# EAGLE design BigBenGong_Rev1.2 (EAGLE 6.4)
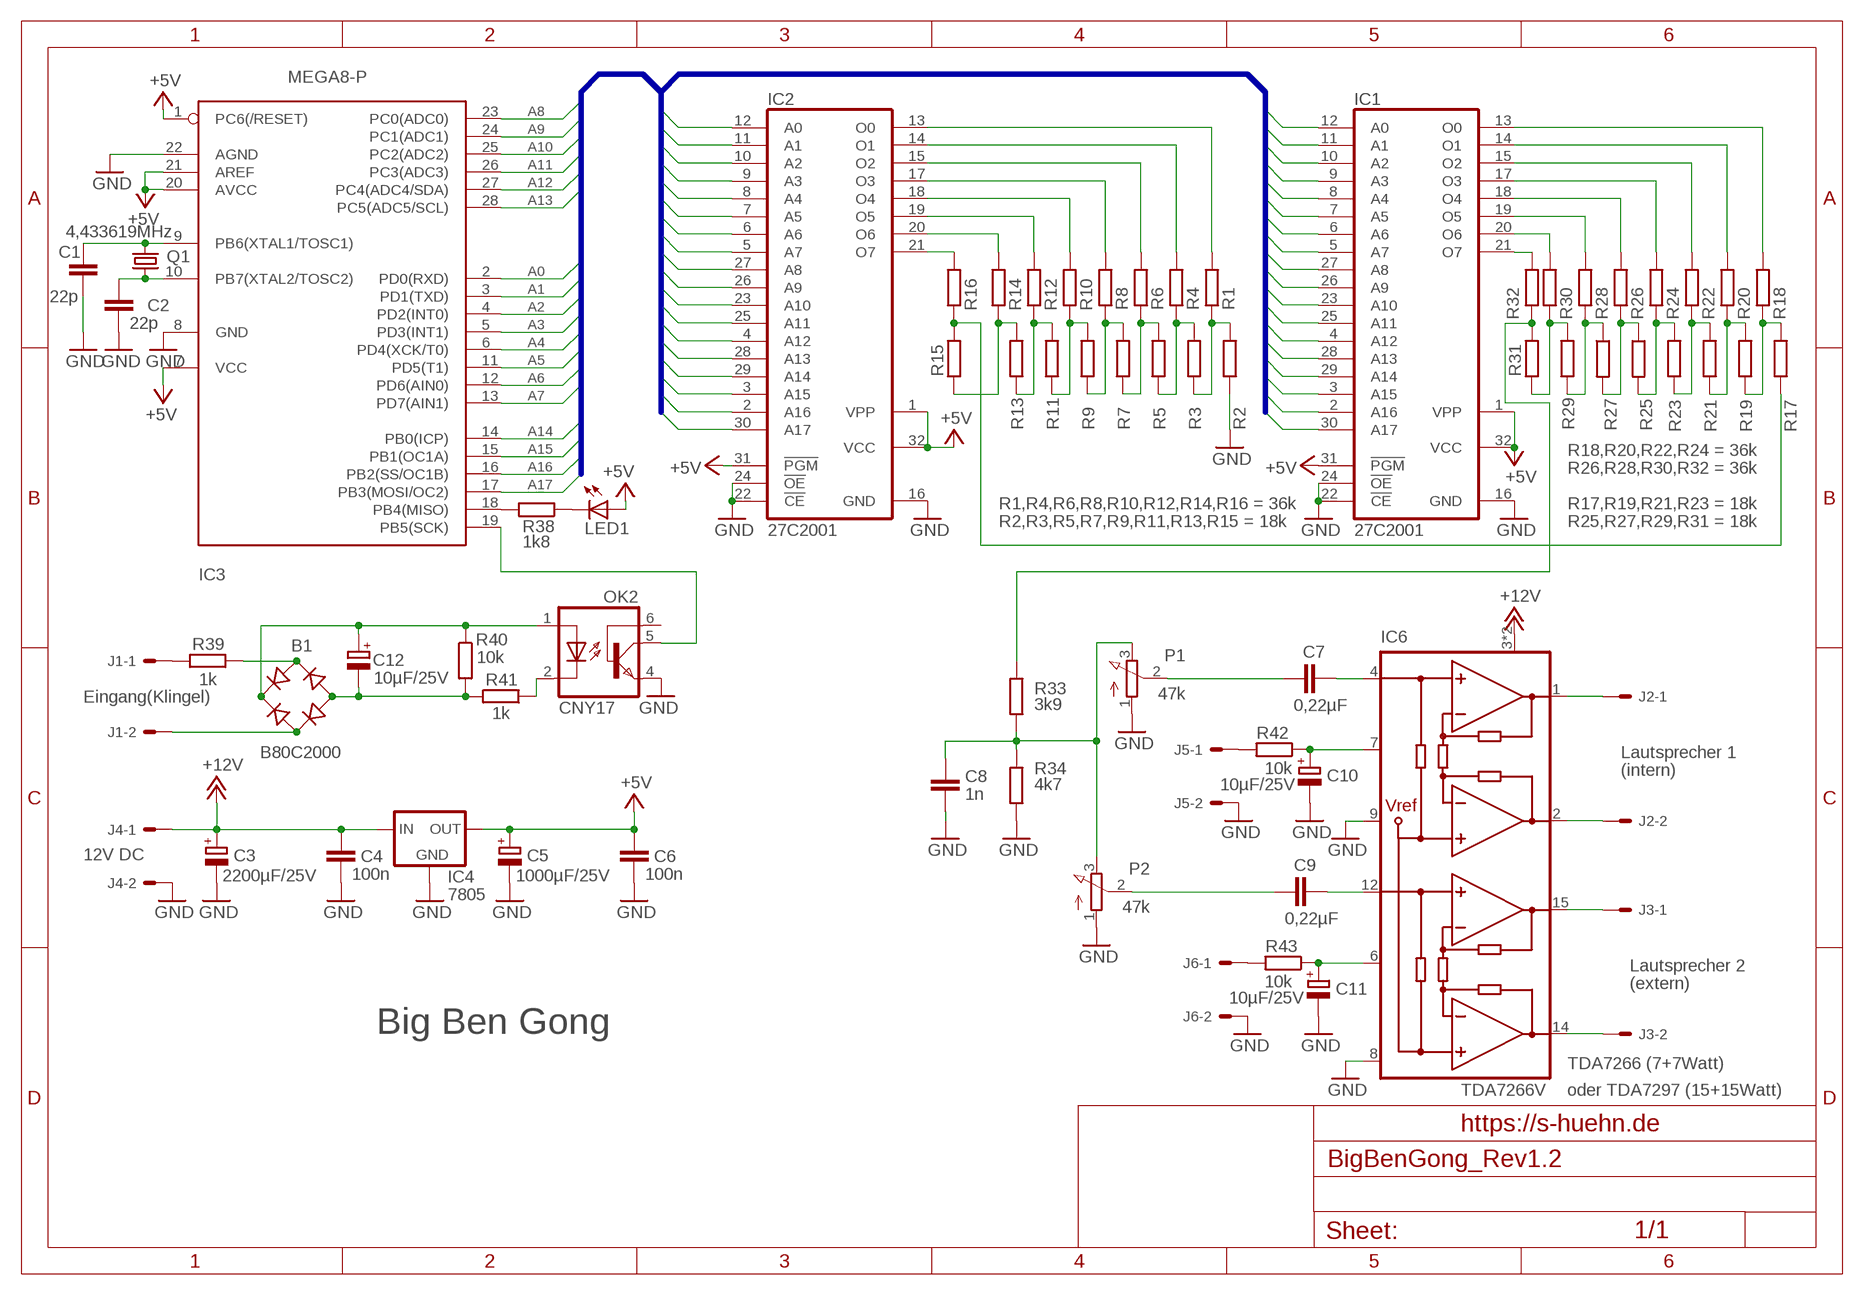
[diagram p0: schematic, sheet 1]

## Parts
B1  B80C2000  RB1A  [RB1A]
C1  22p  C-EU025-25X50A  [C025-025X050A]
C2  22p  C-EU025-25X50A  [C025-025X050A]
C3  2200µF/25V  CPOL-EUE7.5-16  [E7,5-16]
C4  100n  C-EU025-25X50A  [C025-025X050A]
C5  1000µF/25V  CPOL-EUE5-10.5  [E5-10,5]
C6  100n  C-EU025-25X50A  [C025-025X050A]
C7  0,22µF  C-EU025_050-035X075  [C025_050-035X075]
C8  1n  C-EU025-25X50A  [C025-025X050A]
C9  0,22µF  C-EU025_050-035X075  [C025_050-035X075]
C10  10µF/25V  CPOL-EUE2,5-6E  [E2,5-6E]
C11  10µF/25V  CPOL-EUE2,5-6E  [E2,5-6E]
C12  10µF/25V  CPOL-EUE2.5-6  [E2,5-6]
IC1  27C2001  27C2001D  [DIL32]
IC2  27C2001  27C2001D  [DIL32]
IC3  MEGA8-P  [DIL28-3]
IC4  7805  78XXS  [78XXS]
IC6  TDA7266V  [MULTIWATT15V]
J1  22-27-2021-02  [6410-02]
J2  22-27-2021-02  [6410-02]
J3  22-27-2021-02  [6410-02]
J4  22-27-2021-02  [6410-02]
J5  22-27-2021-02  [6410-02]
J6  22-27-2021-02  [6410-02]
LED1  LED5MM_MOLEX_S  [6410-02]
OK2  CNY17  [DIL06]
P1  47k  POTIMOL-H  [6410-03]
P2  47k  POTIMOL-H  [6410-03]
Q1  4,433619MHz  CRYSTALHC49U-V  [HC49U-V]
R1  R-EU_0207/10A  [0207/10A]
R2  R-EU_0207/10A  [0207/10A]
R3  R-EU_0207/10A  [0207/10A]
R4  R-EU_0207/10A  [0207/10A]
R5  R-EU_0207/10A  [0207/10A]
R6  R-EU_0207/10A  [0207/10A]
R7  R-EU_0207/10A  [0207/10A]
R8  R-EU_0207/10A  [0207/10A]
R9  R-EU_0207/10A  [0207/10A]
R10  R-EU_0207/10A  [0207/10A]
R11  R-EU_0207/10A  [0207/10A]
R12  R-EU_0207/10A  [0207/10A]
R13  R-EU_0207/10A  [0207/10A]
R14  R-EU_0207/10A  [0207/10A]
R15  R-EU_0207/10A  [0207/10A]
R16  R-EU_0207/10A  [0207/10A]
R17  R-EU_0207/10A  [0207/10A]
R18  R-EU_0207/10A  [0207/10A]
R19  R-EU_0207/10A  [0207/10A]
R20  R-EU_0207/10A  [0207/10A]
R21  R-EU_0207/10A  [0207/10A]
R22  R-EU_0207/10A  [0207/10A]
R23  R-EU_0207/10A  [0207/10A]
R24  R-EU_0207/10A  [0207/10A]
R25  R-EU_0207/10A  [0207/10A]
R26  R-EU_0207/10A  [0207/10A]
R27  R-EU_0207/10A  [0207/10A]
R28  R-EU_0207/10A  [0207/10A]
R29  R-EU_0207/10A  [0207/10A]
R30  R-EU_0207/10A  [0207/10A]
R31  R-EU_0207/10A  [0207/10A]
R32  R-EU_0207/10A  [0207/10A]
R33  3k9  R-EU_0207/10A  [0207/10A]
R34  4k7  R-EU_0207/10A  [0207/10A]
R38  1k8  R-EU_0207/10A  [0207/10A]
R39  1k  R-EU_0207/10A  [0207/10A]
R40  10k  R-EU_0207/10A  [0207/10A]
R41  1k  R-EU_0207/10A  [0207/10A]
R42  10k  R-EU_0207/10A  [0207/10A]
R43  10k  R-EU_0207/10A  [0207/10A]

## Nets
+5V: C5.+ C6.1 IC1.1(VPP) IC1.31(!PGM) IC1.32(VCC) IC2.1(VPP) IC2.31(!PGM) IC2.32(VCC) IC3.1(PC6(/RESET)) IC3.7(VCC) IC3.20(AVCC) IC3.21(AREF) IC4.OUT LED1.A
+12V: C3.+ C4.1 IC4.IN IC6.3(VCC) IC6.13(VCC) J4.1
A0: IC1.12(A0) IC2.12(A0) IC3.2(PD0(RXD))
A1: IC1.11(A1) IC2.11(A1) IC3.3(PD1(TXD))
A2: IC1.10(A2) IC2.10(A2) IC3.4(PD2(INT0))
A3: IC1.9(A3) IC2.9(A3) IC3.5(PD3(INT1))
A4: IC1.8(A4) IC2.8(A4) IC3.6(PD4(XCK/T0))
A5: IC1.7(A5) IC2.7(A5) IC3.11(PD5(T1))
A6: IC1.6(A6) IC2.6(A6) IC3.12(PD6(AIN0))
A7: IC1.5(A7) IC2.5(A7) IC3.13(PD7(AIN1))
A8: IC1.27(A8) IC2.27(A8) IC3.23(PC0(ADC0))
A9: IC1.26(A9) IC2.26(A9) IC3.24(PC1(ADC1))
A10: IC1.23(A10) IC2.23(A10) IC3.25(PC2(ADC2))
A11: IC1.25(A11) IC2.25(A11) IC3.26(PC3(ADC3))
A12: IC1.4(A12) IC2.4(A12) IC3.27(PC4(ADC4/SDA))
A13: IC1.28(A13) IC2.28(A13) IC3.28(PC5(ADC5/SCL))
A14: IC1.29(A14) IC2.29(A14) IC3.14(PB0(ICP))
A15: IC1.3(A15) IC2.3(A15) IC3.15(PB1(OC1A))
A16: IC1.2(A16) IC2.2(A16) IC3.16(PB2(SS/OC1B))
A17: IC1.30(A17) IC2.30(A17) IC3.17(PB3(MOSI/OC2))
GND: C1.2 C2.2 C3.- C4.2 C5.- C6.2 C8.2 C10.- C11.- IC1.16(GND) IC1.22(!CE) IC1.24(!OE) IC2.16(GND) IC2.22(!CE) IC2.24(!OE) IC3.8(GND) IC3.22(AGND) IC4.GND IC6.8(PW-GND) IC6.9(S-GND) J4.2 J5.2 J6.2 OK2.4(EMI) P1.1(A) P2.1(A) R2.1 R34.2
N$1: IC2.13(O0) R1.1
N$2: IC2.14(O1) R4.1
N$3: IC2.17(O3) R8.1
N$4: IC2.18(O4) R10.1
N$5: IC2.15(O2) R6.1
N$6: IC2.19(O5) R12.1
N$7: IC2.20(O6) R14.1
N$8: IC2.21(O7) R16.1
N$9: IC1.13(O0) R18.1
N$10: IC1.14(O1) R20.1
N$11: IC1.15(O2) R22.1
N$12: IC1.17(O3) R24.1
N$13: IC1.18(O4) R26.1
N$14: IC1.19(O5) R28.1
N$15: IC1.20(O6) R30.1
N$16: IC1.21(O7) R32.1
N$17: B1.+ C12.+ OK2.1(A) R40.1
N$18: R29.2 R30.2 R31.1
N$19: R27.1 R28.2 R29.1
N$20: R25.1 R26.2 R27.2
N$21: R23.2 R24.2 R25.2
N$22: R21.2 R22.2 R23.1
N$23: R19.2 R20.2 R21.1
N$24: R17.2 R18.2 R19.1
N$25: R15.2 R16.2 R17.1
N$26: R13.2 R14.2 R15.1
N$27: C1.1 IC3.9(PB6(XTAL1/TOSC1)) Q1.2
N$28: R11.2 R12.2 R13.1
N$29: C2.1 IC3.10(PB7(XTAL2/TOSC2)) Q1.1
N$30: R9.2 R10.2 R11.1
N$31: R7.2 R8.2 R9.1
N$32: R5.2 R6.2 R7.1
N$33: R3.2 R4.2 R5.1
N$34: R1.2 R2.2 R3.1
N$35: IC3.18(PB4(MISO)) R38.2
N$36: IC3.19(PB5(SCK)) OK2.5(COL)
N$37: OK2.2(C) R41.1
N$38: B1.- C12.- R40.2 R41.2
N$41: C7.1 IC6.4(IN1)
N$42: R31.2 R32.2 R33.1
N$43: LED1.C R38.1
N$44: J1.1 R39.1
N$45: B1.AC2 J1.2
N$46: IC6.1(OUT1+) J2.1
N$47: IC6.2(OUT1-) J2.2
N$48: IC6.15(OUT2+) J3.1
N$49: IC6.14(OUT2-) J3.2
N$50: C9.1 IC6.12(IN2)
N$51: B1.AC1 R39.2
N$52: C10.+ IC6.7(ST-BY) R42.1
N$53: C11.+ IC6.6(MUTE) R43.1
N$54: J5.1 R42.2
N$55: J6.1 R43.2
N$56: C7.2 C7.3 P1.2(S)
N$57: C9.2 C9.3 P2.2(S)
N$58: C8.1 P1.3(E) P2.3(E) R33.2 R34.1
Unconnected: OK2.6(BAS)

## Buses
A[0..17]

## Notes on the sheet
- R18,R20,R22,R24 = 36k
- R26,R28,R30,R32 = 36k
- R1,R4,R6,R8,R10,R12,R14,R16 = 36k | R17,R19,R21,R23 = 18k
- R2,R3,R5,R7,R9,R11,R13,R15 = 18k | R25,R27,R29,R31 = 18k
- Eingang(Klingel)
- Lautsprecher 1
- (intern)
- 12V DC
- Lautsprecher 2
- (extern)
- Big Ben Gong
- TDA7266 (7+7Watt)
- oder TDA7297 (15+15Watt)
- https://s-huehn.de

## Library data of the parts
B1 = rectifier:RB1A: RECTIFIER 1 A
C1 C2 C4 C6-C9 = rcl:C-EU: CAPACITOR, European symbol
C3 C5 C10-C12 = rcl:CPOL-EU: POLARIZED CAPACITOR, European symbol
IC1 IC2 = memory-nec:27C2001D: MEMORY
IC3 = avr-7:MEGA8-P: MICROCONTROLLER 8 Kbytes FLASH 1 kbytes SRAM 512 bytes EEPROM USART 4-channel 10 bit ADC 2-channel 8 bit ADC
IC4 = v-reg:78XXS: VOLTAGE REGULATOR
IC6 = sgs-thom:TDA7266
J1-J6 = con-molex:22-?-02: CONNECTOR
LED1 = led:LED: LED
OK2 = optocoupler-2:CNY17: SIEMENS OPTO COUPLER
P1 P2 = pot:POTI
Q1 = crystal:CRYSTAL: CRYSTAL
R1-R34 R38-R43 = rcl:R-EU_: RESISTOR, European symbol

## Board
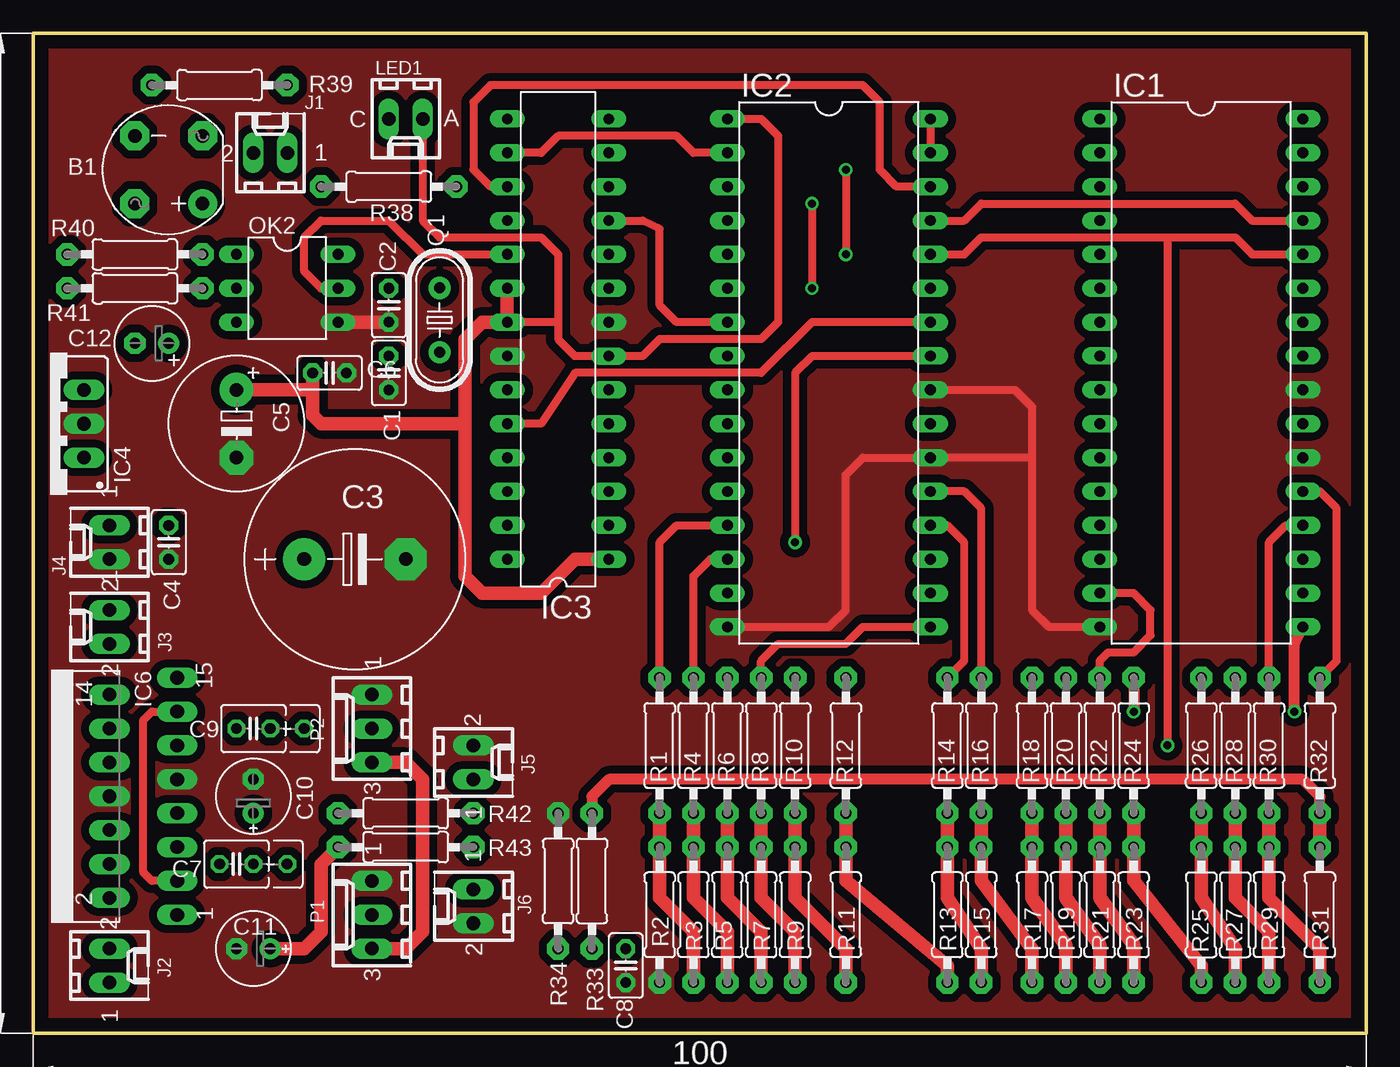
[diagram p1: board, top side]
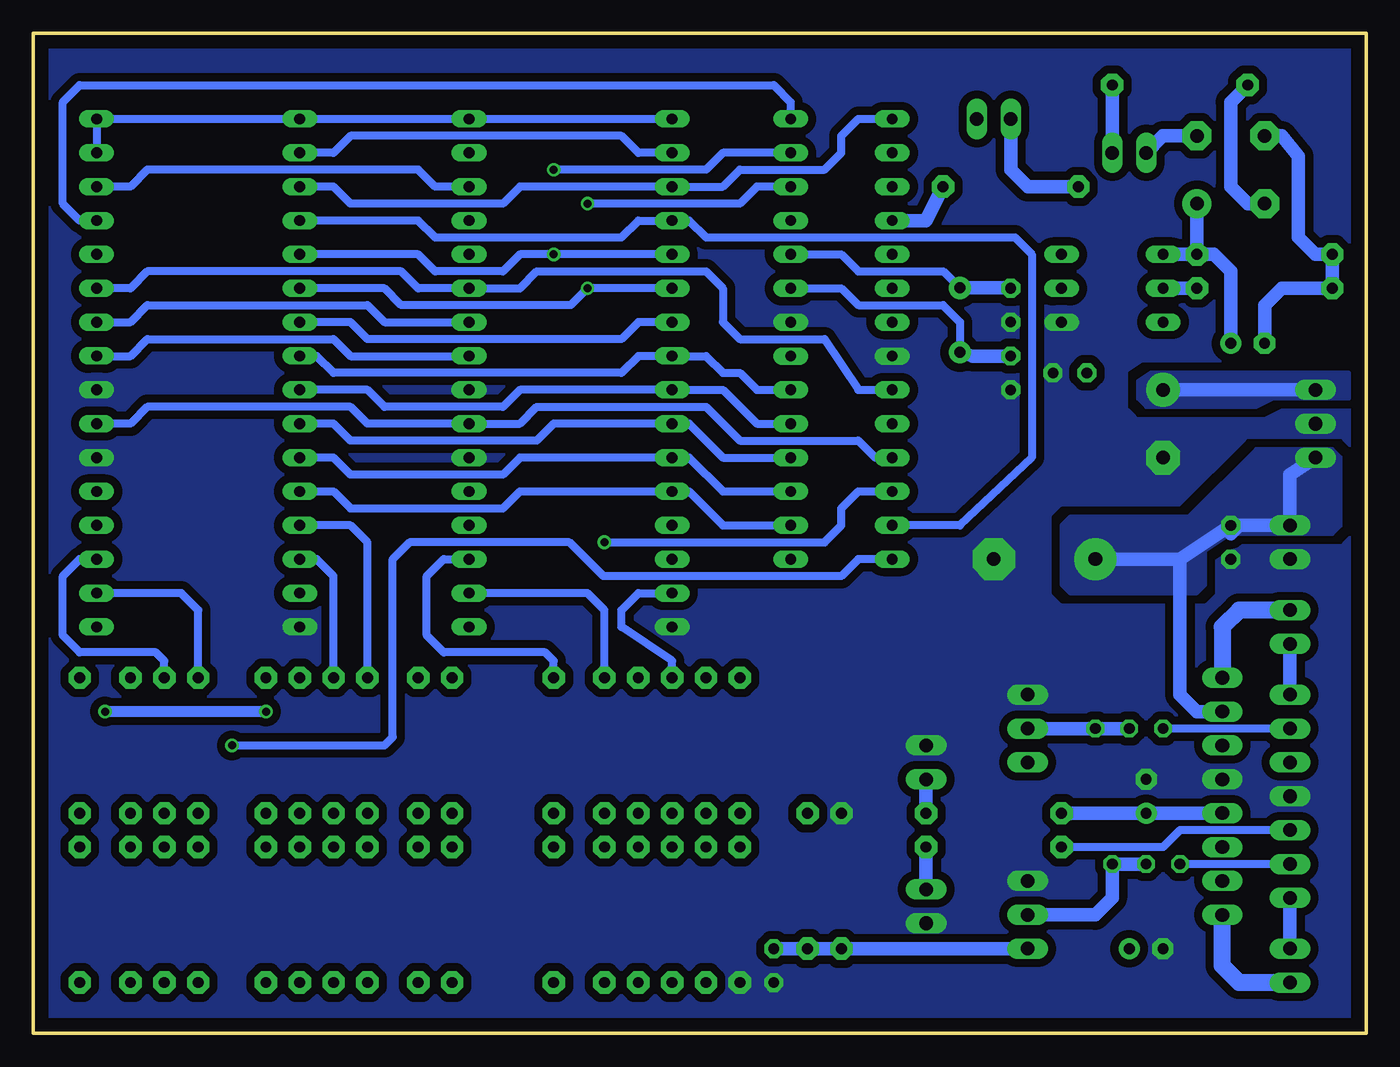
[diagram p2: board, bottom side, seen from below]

Size 100 x 75 mm. Coordinates in mm from the lower left corner, seen from the top.
Outline: 0,0 100,0 100,75 0,75 0,0
Copper layers (1*16): Top 0.035mm / dielectric 1.5mm / Bottom 0.035mm
Design rules "default *": minimum track width 10mil, minimum drill 0.2mm, track to track 8mil, track to pad 8mil, pad to pad 8mil, via to via 8mil, smd to smd 8mil, copper to edge 40mil, drill to drill 8mil, minimum pad ring 10mil, minimum via ring 8mil, stop-mask expansion 4mil, vias tented up to drill 0mil, thermal gap 10mil

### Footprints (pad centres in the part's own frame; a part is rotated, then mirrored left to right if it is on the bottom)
RB1A = drill 1.016 pad 2.184: + -2.54,2.54 | drill 1.016 pad 2.184 octagon: - 2.54,-2.54; AC1 2.54,2.54; AC2 -2.54,-2.54
C025-025X050A = drill 0.8 pad 1.422 octagon: 1 -1.27,0; 2 1.27,0
E7,5-16 = drill 1.016 pad 3.15: + -3.81,0 | drill 1.016 pad 3.15 octagon: - 3.81,0
E5-10,5 = drill 1.016 pad 2.54: + -2.54,0 | drill 1.016 pad 2.54 octagon: - 2.54,0
C025_050-035X075 = drill 0.813 octagon: 1 -1.27,0; 2 1.27,0; 3 3.81,0
E2,5-6E = drill 0.813 pad 1.575: + -1.27,0 | drill 0.813 pad 1.575 octagon: - 1.27,0
E2,5-6 = drill 0.813 pad 1.6: + -1.27,0 | drill 0.813 pad 1.6 octagon: - 1.27,0
DIL32 = drill 0.813 long: 1 -19.05,-7.62; 2 -16.51,-7.62; 3 -13.97,-7.62; 4 -11.43,-7.62; 5 -8.89,-7.62; 6 -6.35,-7.62; 7 -3.81,-7.62; 8 -1.27,-7.62; 9 1.27,-7.62; 10 3.81,-7.62; 11 6.35,-7.62; 12 8.89,-7.62; 13 11.43,-7.62; 14 13.97,-7.62; 15 16.51,-7.62; 16 19.05,-7.62; 17 19.05,7.62; 18 16.51,7.62; 19 13.97,7.62; 20 11.43,7.62; 21 8.89,7.62; 22 6.35,7.62; 23 3.81,7.62; 24 1.27,7.62; 25 -1.27,7.62; 26 -3.81,7.62; 27 -6.35,7.62; 28 -8.89,7.62; 29 -11.43,7.62; 30 -13.97,7.62; 31 -16.51,7.62; 32 -19.05,7.62
DIL28-3 = drill 0.813 long: 1 -16.51,-3.81; 2 -13.97,-3.81; 3 -11.43,-3.81; 4 -8.89,-3.81; 5 -6.35,-3.81; 6 -3.81,-3.81; 7 -1.27,-3.81; 8 1.27,-3.81; 9 3.81,-3.81; 10 6.35,-3.81; 11 8.89,-3.81; 12 11.43,-3.81; 13 13.97,-3.81; 14 16.51,-3.81; 15 16.51,3.81; 16 13.97,3.81; 17 11.43,3.81; 18 8.89,3.81; 19 6.35,3.81; 20 3.81,3.81; 21 1.27,3.81; 22 -1.27,3.81; 23 -3.81,3.81; 24 -6.35,3.81; 25 -8.89,3.81; 26 -11.43,3.81; 27 -13.97,3.81; 28 -16.51,3.81
78XXS = drill 1.016 long: GND 0,-2.54; IN -2.54,-2.54; OUT 2.54,-2.54
MULTIWATT15V = drill 1.016 long: 1 -8.89,-7.62; 2 -7.62,-2.54; 3 -6.35,-7.62; 4 -5.08,-2.54; 5 -3.81,-7.62; 6 -2.54,-2.54; 7 -1.27,-7.62; 8 0,-2.54; 9 1.27,-7.62; 10 2.54,-2.54; 11 3.81,-7.62; 12 5.08,-2.54; 13 6.35,-7.62; 14 7.62,-2.54; 15 8.89,-7.62
6410-02 = drill 1.016 long: 1 1.27,0; 2 -1.27,0
6410-02' = drill 1.016 long: A -1.27,0; C 1.27,0
DIL06 = drill 0.813 long: 1 -2.54,-3.81; 2 0,-3.81; 3 2.54,-3.81; 4 2.54,3.81; 5 0,3.81; 6 -2.54,3.81
6410-03 = drill 1.016 long: 1 2.54,0; 2 0,0; 3 -2.54,0
HC49U-V = drill 0.813 pad 1.676: 1 -2.413,0; 2 2.413,0
0207/10A = drill 0.813 pad 1.676 octagon: 1 -5.08,0; 2 5.08,0

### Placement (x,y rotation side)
B1  10.16,64.77 180 top
C1  26.67,49.53 270 top
C2  26.67,54.61 270 top
C3  24.13,35.56 0 top
C4  10.16,36.83 270 top
C5  15.24,45.72 270 top
C6  22.23,49.53 0 top
C7  15.24,12.7 0 top
C8  44.45,5.08 270 top
C9  16.51,22.86 0 top
C10  16.51,17.78 90 top
C11  16.51,6.35 180 top
C12  8.89,51.75 180 top
IC1  87.63,49.53 270 top
IC2  59.69,49.53 270 top
IC3  39.37,52.07 90 top
IC4  1.27,45.72 90 top
IC6  3.17,17.78 90 top
J1  17.78,66.04 0 top
J2  5.71,5.08 270 top
J3  5.71,30.48 90 top
J4  5.71,36.83 90 top
J5  33.02,20.32 270 top
J6  33.02,9.53 90 top
LED1  [6410-02']  27.94,68.58 180 top
OK2  19.05,55.88 270 top
P1  25.4,8.89 90 top
P2  25.4,22.86 90 top
Q1  30.48,53.5 270 top
R1  46.99,21.59 270 top
R2  46.99,8.89 90 top
R3  49.53,8.89 90 top
R4  49.53,21.59 270 top
R5  52.07,8.89 90 top
R6  52.07,21.59 270 top
R7  54.61,8.89 90 top
R8  54.61,21.59 270 top
R9  57.15,8.89 90 top
R10  57.15,21.59 270 top
R11  60.96,8.89 90 top
R12  60.96,21.59 270 top
R13  68.58,8.89 90 top
R14  68.58,21.59 270 top
R15  71.12,8.89 90 top
R16  71.12,21.59 270 top
R17  74.93,8.89 90 top
R18  74.93,21.59 270 top
R19  77.47,8.89 90 top
R20  77.47,21.59 270 top
R21  80.01,8.89 90 top
R22  80.01,21.59 270 top
R23  82.55,8.89 90 top
R24  82.55,21.59 270 top
R25  87.63,8.89 270 top
R26  87.63,21.59 270 top
R27  90.17,8.89 270 top
R28  90.17,21.59 270 top
R29  92.71,8.89 90 top
R30  92.71,21.59 270 top
R31  96.52,8.89 90 top
R32  96.52,21.59 270 top
R33  41.91,11.43 270 top
R34  39.37,11.43 90 top
R38  26.67,63.5 0 top
R39  13.97,71.12 180 top
R40  7.62,58.42 180 top
R41  7.62,55.88 180 top
R42  27.94,16.51 0 top
R43  27.94,13.97 0 top

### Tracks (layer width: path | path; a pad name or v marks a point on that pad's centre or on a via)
+5V
  Top 0.61: IC2.32 IC2.31 | IC2.1 54.61,68.58 55.88,67.31 55.88,53.34 54.61,52.07 46.99,52.07 45.72,50.8 IC3.7 40.64,50.8 39.37,52.07 39.37,53.34 | 39.37,53.34 IC3.21 | LED1.A 29.21,60.96 30.48,59.69 38.1,59.69 39.37,58.42 39.37,53.34
  Top 1.016: IC3.20 IC3.21 33.66,53.34 32.38,52.07 32.38,45.72 | 32.38,45.72 32.38,34.29 33.66,33.02 38.1,33.02 40.64,35.56 IC3.1 | 32.38,45.72 21.59,45.72 20.95,46.35 20.95,48.26 | 20.95,48.26 C5.+ | C6.1 20.95,48.26
  Bottom 0.61: IC2.1 IC2.32 IC1.1 IC1.32 IC1.31
  Bottom 1.016: IC4.OUT C5.+
  pour Bottom (rank 2, no thermals): 1.27,49.53 16.19,49.53 17.14,48.9 17.14,47.62 16.51,46.99 8.26,46.99 6.99,47.62 1.27,47.62
+12V
  Top 0.61: IC6.3 8.89,11.43 8.26,12.06 8.26,23.5 8.89,24.13 IC6.13
  Bottom 1.016: IC4.IN 5.71,41.91 J4.1 9.53,38.1 10.16,37.47 C4.1 13.97,35.56 | 13.97,35.56 13.97,25.4 12.7,24.13 IC6.13 | C3.+ 13.97,35.56
  pour Bottom (rank 2, no thermals): 2.54,43.81 8.26,43.81 13.34,38.73 22.23,38.73 22.86,38.1 22.86,33.66 22.23,33.02 12.7,33.02 12.06,33.66 12.06,36.2 10.16,37.47 2.54,37.47 1.91,38.1 1.91,43.18
A0
  Bottom 0.254: IC2.12 50.8,40.64
  Bottom 0.61: IC2.12 63.5,40.64 64.77,39.37 76.2,39.37 77.47,40.64 IC1.12 | 50.8,40.64 48.26,38.1 IC3.2
A1
  Bottom 0.61: IC3.3 48.26,40.64 50.8,43.18 IC2.11 63.5,43.18 64.77,41.91 76.2,41.91 77.47,43.18 IC1.11
A2
  Bottom 0.254: IC2.10 50.8,45.72
  Bottom 0.61: IC3.4 48.26,43.18 50.8,45.72 | IC1.10 77.47,45.72 76.2,44.45 62.23,44.45 60.96,45.72 IC2.10
A3
  Bottom 0.61: IC1.9 74.93,48.26 73.66,46.99 64.77,46.99 63.5,48.26 IC2.9 48.26,48.26 45.72,45.72 IC3.5
A4
  Bottom 0.61: IC1.8 78.74,50.8 77.47,49.53 55.88,49.53 54.61,50.8 IC2.8 49.53,50.8 48.26,49.53 46.99,49.53 45.72,48.26 IC3.6
A5
  Top 0.61: IC3.11 45.72,60.96 46.99,60.33 46.99,54.61 48.26,53.34 IC2.7
  Bottom 0.61: IC1.7 76.2,53.34 74.93,52.07 55.88,52.07 54.61,53.34 IC2.7
A6  (via drill 0.6)
  Top 0.61: v58.42,62.23 v58.42,55.88
  Bottom 0.61: IC1.6 73.66,55.88 72.39,54.61 59.69,54.61 v58.42,55.88 IC2.6 | IC3.12 45.72,63.5 46.99,62.23 v58.42,62.23
A7  (via drill 0.6)
  Top 0.61: v60.96,64.77 v60.96,58.42
  Bottom 0.61: IC1.5 71.12,58.42 69.85,57.15 64.77,57.15 63.5,58.42 v60.96,58.42 IC2.5 | IC3.13 48.26,66.04 49.53,64.77 v60.96,64.77
A8
  Bottom 0.61: IC1.27 92.71,55.88 91.44,57.15 72.39,57.15 71.12,55.88 IC2.27 63.5,55.88 62.23,57.15 49.53,57.15 48.26,55.88 48.26,53.34 46.99,52.07 40.64,52.07 38.1,48.26 IC3.23
A9
  Top 0.61: IC3.24 38.1,45.72 40.64,49.53 54.61,49.53 58.42,53.34 IC2.26
  Bottom 0.61: IC2.26 73.66,53.34 74.93,54.61 91.44,54.61 92.71,53.34 IC1.26
A10
  Bottom 0.61: IC3.25 36.83,43.18 38.1,44.45 46.99,44.45 49.53,46.99 62.23,46.99 63.5,45.72 IC2.23 74.93,45.72 76.2,46.99 91.44,46.99 92.71,45.72 IC1.23
A11  (via drill 0.61)
  Top 0.61: v57.15,36.83 57.15,49.53 58.42,50.8 IC2.25
  Bottom 0.61: IC2.25 76.2,50.8 77.47,52.07 91.44,52.07 92.71,50.8 IC1.25 | IC3.26 38.1,40.64 39.37,39.37 39.37,38.1 40.64,36.83 v57.15,36.83
A12
  Bottom 0.61: IC1.4 71.12,60.96 69.85,59.69 55.88,59.69 54.61,60.96 IC2.4 50.8,60.96 49.53,59.69 26.35,59.69 25.08,58.42 25.08,43.18 30.48,38.1 IC3.27
A13  (via drill 0.6)
  Top 0.61: IC1.28 91.44,58.42 90.17,59.69 85.09,59.69 | IC2.28 69.85,58.42 71.12,59.69 85.09,59.69 | 85.09,59.69 v85.09,21.59
  Bottom 0.61: IC3.28 38.1,35.56 39.37,34.29 57.23,34.29 59.77,36.83 71.75,36.83 73.03,35.56 73.03,22.23 73.66,21.59 v85.09,21.59
A14
  Top 0.61: IC1.29 91.44,60.96 90.17,62.23 71.12,62.23 69.85,60.96 IC2.29
  Bottom 0.61: IC3.14 43.18,69.85 44.45,71.12 96.52,71.12 97.79,69.85 97.79,62.23 96.52,60.96 IC1.29
A15
  Bottom 0.61: IC1.3 77.47,63.5 76.2,62.23 64.77,62.23 63.5,63.5 IC2.3 48.26,63.5 46.99,64.77 40.64,64.77 39.37,66.04 39.37,67.31 38.1,68.58 IC3.15
A16
  Top 0.61: IC3.16 38.1,66.04 39.37,67.31 48.26,67.31 49.53,66.04 IC2.2
  Bottom 0.61: IC1.2 77.47,66.04 76.2,67.31 55.88,67.31 54.61,66.04 IC2.2
A17
  Top 0.61: IC3.17 34.29,63.5 33.02,64.77 33.02,69.85 34.29,71.12 62.23,71.12 63.5,69.85 63.5,64.77 64.77,63.5 IC2.30
  Bottom 0.254: IC2.30 68.58,63.5
  Bottom 0.61: IC1.30 92.71,63.5 91.44,64.77 71.12,64.77 69.85,63.5 68.58,63.5
GND
  Top 0.61: IC2.24 73.66,48.26 74.93,46.99 74.93,43.18 | 74.93,43.18 IC2.22 62.23,43.18 60.96,41.91 60.96,31.75 59.69,30.48 IC2.16 | 74.93,43.18 74.93,31.75 76.2,30.48 IC1.16
  Top 1.016: OK2.4 C2.2
  Bottom 0.254: IC2.22
  pour Top (isolate 0.61, no thermals): 0,0 100,0 100,2 100,75 0,75 0,64
  pour Bottom (isolate 0.61, rank 6, no thermals): 0,0 100,0 100,2 100,75 0,75 0,71
N$1
  Top 0.61: IC2.13 48.26,38.1 46.99,36.83 R1.1
N$2
  Top 0.61: IC2.14 50.8,35.56 49.53,34.29 R4.1
N$3
  Top 0.61: IC2.17 62.23,30.48 60.96,29.21 55.88,29.21 54.61,27.94 R8.1
N$4
  Bottom 0.61: IC2.18 58.42,33.02 57.15,31.75 R10.1
N$5
  Bottom 0.61: IC2.15 54.61,33.02 55.88,31.75 55.88,30.48 52.07,27.94 R6.1
N$6
  Bottom 0.61: IC2.19 69.22,35.56 70.48,34.29 70.48,29.84 69.22,28.57 61.59,28.57 60.96,27.94 R12.1
N$7
  Top 0.61: IC2.20 68.58,38.1 69.85,36.83 69.85,27.94 R14.1
N$8
  Top 0.61: IC2.21 69.85,40.64 71.12,39.37 R16.1
N$9
  Bottom 0.61: IC1.13 76.2,38.1 74.93,36.83 R18.1
N$10
  Bottom 0.61: IC1.14 78.74,35.56 77.47,34.29 R20.1
N$11
  Top 0.61: IC1.15 82.55,33.02 83.82,31.75 83.82,29.84 82.55,28.57 80.64,28.57 80.01,27.94 R22.1
N$12  (via drill 0.6)
  Top 0.813: v94.61,24.13 94.61,29.21 IC1.17 | R24.1 v82.55,24.13
  Bottom 0.813: v82.55,24.13 v94.61,24.13
N$13
  Bottom 0.61: IC1.18 88.9,33.02 87.63,31.75 R26.1
N$14
  Bottom 0.61: IC1.19 96.52,35.56 97.79,34.29 97.79,29.84 96.52,28.57 90.81,28.57 90.17,27.94 R28.1
N$15
  Top 0.61: IC1.20 93.98,38.1 92.71,36.83 R30.1
N$16
  Top 0.61: IC1.21 96.52,40.64 97.79,39.37 97.79,27.94 R32.1
N$17
  Bottom 1.016: B1.+ R40.1 | R40.1 OK2.1 | C12.+ 10.16,57.15 11.43,58.42 R40.1
N$18
  Top 1.016: R30.2 R29.2 92.71,10.16 96.52,6.35 R31.1
N$19
  Top 1.016: R28.2 R27.1 90.17,10.16 92.71,7.62 R29.1
N$20
  Top 1.016: R26.2 R25.1 87.63,10.16 90.17,6.35 R27.2
N$21
  Top 1.016: R24.2 R23.2 82.55,11.43 87.63,5.08 R25.2
N$22
  Top 1.016: R22.2 R21.2 80.01,10.16 82.55,6.62 R23.1
N$23
  Top 1.016: R20.2 R19.2 77.47,10.16 80.01,6.62 R21.1
N$24
  Top 1.016: R18.2 R17.2 74.93,10.16 77.47,6.62 R19.1
N$25
  Top 1.016: R16.2 R15.2 71.12,11.43 74.93,6.35 R17.1
N$26
  Top 1.016: R14.2 R13.2 68.58,10.16 71.12,6.35 R15.1
N$27
  Bottom 0.61: IC3.9 39.37,55.88 38.1,54.61 31.75,54.61 30.48,53.34 Q1.2
  Bottom 1.016: Q1.2 29.49,50.77 C1.1
N$28
  Top 1.016: R12.2 R11.2 60.96,11.43 68.58,5.08 R13.1
N$29
  Bottom 0.61: 26.7,55.91 C2.1 | IC3.10 39.37,58.42 38.1,57.15 31.72,57.15 Q1.1
  Bottom 1.016: Q1.1 26.7,55.91
N$30
  Top 1.016: R10.2 R9.2 57.15,10.16 60.96,6.35 R11.1
N$31
  Top 1.016: R8.2 R7.2 54.61,10.16 57.15,7.62 R9.1
N$32
  Top 1.016: R6.2 R5.2 52.07,10.16 54.61,7.62 R7.1
N$33
  Top 1.016: R4.2 R3.2 49.53,10.16 52.07,7.62 R5.1
N$34
  Top 1.016: R1.2 R2.2 46.99,10.16 49.53,7.62 R3.1
N$35
  Bottom 1.016: R38.2 33.02,60.96 IC3.18
N$36
  Top 0.61: OK2.5 21.59,55.88 20.32,57.15 20.32,59.69 21.59,60.96 26.67,60.96 29.21,58.42 IC3.19
N$37
  Bottom 1.016: R41.1 OK2.2
N$38
  Bottom 1.016: B1.- 6.35,67.31 5.08,65.77 5.08,59.69 3.81,58.42 R40.2 R41.2 6.35,55.88 7.62,54.61 C12.-
N$41
  Bottom 0.61: IC6.4 C7.1
N$42
  Top 0.813: R32.2 96.52,17.78 95.25,19.05 43.18,19.05 41.91,17.78 R33.1
  Top 1.016: R32.2 R31.2
N$43
  Bottom 1.016: R38.1 25.4,63.5 26.67,64.77 LED1.C
N$44
  Bottom 1.016: R39.1 J1.1
N$45
  Bottom 1.016: J1.2 15.24,67.31 B1.AC2
N$46
  Bottom 1.27: J2.1 9.53,3.81 10.79,5.08 IC6.1
N$47
  Bottom 1.016: IC6.2 J2.2
N$48
  Bottom 1.27: J3.1 9.53,31.75 10.79,30.48 IC6.15
N$49
  Bottom 1.016: J3.2 IC6.14
N$50
  Bottom 0.61: IC6.12 C9.1
N$51
  Bottom 1.016: R39.2 10.16,69.85 10.16,63.5 8.89,62.23 B1.AC1
N$52
  Bottom 1.016: R42.1 C10.+ IC6.7
N$53
  Top 1.016: C11.+ 20.32,6.35 21.59,7.62 21.59,12.7 R43.1
  Bottom 0.61: IC6.6 13.97,15.24 15.24,13.97 R43.1
N$54
  Bottom 1.016: R42.2 J5.1
N$55
  Bottom 1.016: R43.2 J6.1
N$56
  Bottom 1.016: C7.2 C7.3 19.05,10.16 20.32,8.89 P1.2
N$57
  Bottom 1.016: C9.2 C9.3 P2.2
N$58
  Top 1.016: P1.3 27.94,6.35 29.21,7.62 29.21,19.05 27.94,20.32 P2.3
  Bottom 1.016: C8.1 R33.2 R34.1 P1.3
